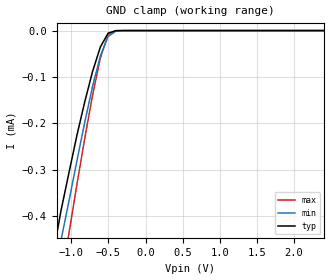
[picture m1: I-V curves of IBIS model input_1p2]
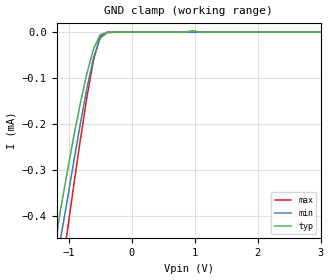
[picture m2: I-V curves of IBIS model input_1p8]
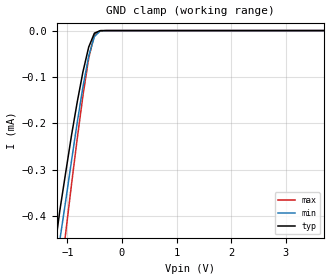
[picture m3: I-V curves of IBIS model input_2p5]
| Texas Instruments Incorporated
| SN74LXC2T45 2-Bit Dual Supply Voltage Translator
| with 3-State outputs and Schmitt-trigger Inputs
[IBIS Ver]   4.1
[File name]   sn74lxc2t45.ibs
[File Rev]   1.0
[Date]   04/24/2019
[Source]
| Texas Instruments Incorporated.
| Analog-eLab Design Center, HPA
| 12500 TI Blvd
| Dallas, TX -75243
[Notes]   Revision History:
| Rev 1.0: 09/01/2020
| - Initial version of the model
| - Model generated from simulations in SPECTRE
| - C_comp although listed in numerical order of value are
|   obtained from varying PVT conditions. For PVT conditions for
|   each specific value refer the buffer description under
|   respective [Model]. IBIS model user is responsible for using
|   appropriate C_comp to simulate for Signal Integrity.
| - Warnings regarding combined Non-monotonicity of various models have been
|   reviewd and considered minor and can be ignored.
| - Model names with a trailing _2p5 contain the model for 2.5V operation.
[Disclaimer]
| This model is designed as an aid for customers of Texas Instruments.
| TI and its licensors and suppliers make no warranties, either expressed
| or implied, with respect to this  model, including the warranties of
| merchantability or fitness for a particular purpose. The model is
| provided solely on an "as is" basis. The entire risk as to its quality
| and performance is with the customer.
| This model is subject to change without notice. Texas Instruments
| Incorporated is not responsible for updating this model.
[Copyright]
 (C) Copyright 2020 Texas Instruments Incorporated.All rights reserved.
| Component LXC2T45_DCT 8-pin SOT
[Component]   SN74LXC2T45DCT
[Manufacturer]   Texas Instruments, Inc.
[Package]
|   typ   min   max
R_pkg   2.900e-02   2.800e-02   3.100e-02
L_pkg   1.796e-09   1.666e-09   1.924e-09
C_pkg   2.310e-13   2.210e-13   2.420e-13
[Pin]   signal_name   model_name   R_pin   L_pin   C_pin
1   VCCA   power   3.100e-02   1.894e-09   2.230e-13
2   A1   I/O   2.800e-02   1.697e-09   2.370e-13
3   A2   I/O   3.000e-02   1.722e-09   2.390e-13
4   GND   gnd   3.000e-02   1.861e-09   2.210e-13
5   DIR   input   2.800e-02   1.924e-09   2.280e-13
6   B2   I/O   2.900e-02   1.736e-09   2.420e-13
7   B1   I/O   2.800e-02   1.666e-09   2.360e-13
8   VCCB   power   3.000e-02   1.871e-09   2.220e-13
| Component LXC2T45_DCU 8-pin SOT
[Component]   SN74LXC2T45DCU
[Manufacturer]   Texas Instruments, Inc.
[Package]
|   typ   min   max
R_pkg   2.600e-02   2.300e-02   3.800e-02
L_pkg   1.394e-09   1.066e-09   2.046e-09
C_pkg   2.590e-13   2.150e-13   3.720e-13
[Pin]   signal_name   model_name   R_pin   L_pin   C_pin
1   VCCA   power   2.400e-02   1.520e-09   2.710e-13
2   A1   I/O   2.300e-02   1.112e-09   2.180e-13
3   A2   I/O   2.300e-02   1.070e-09   2.170e-13
4   GND   gnd   2.700e-02   2.046e-09   3.720e-13
5   DIR   input   2.700e-02   1.542e-09   2.730e-13
6   B2   I/O   2.300e-02   1.100e-09   2.240e-13
7   B1   I/O   2.300e-02   1.066e-09   2.150e-13
8   VCCB   power   3.800e-02   1.696e-09   2.800e-13
|Component
[Component]   SN74LXC2T45DTM
[Manufacturer]  TI
[Package]   |  8 pin  X2SON
|   typ   min   max
R_pkg   0.05   0.04   0.06
L_pkg   1.0nH   0.8nH   1.2nH
C_pkg   0.2pF   0.16pF   0.24pF
[Pin]  signal_name model_name   R_pin   L_pin   C_pin
1   VCCA   power   NA   NA   NA
2   A1   I/O   NA   NA   NA
3   A2   I/O   NA   NA   NA
4   GND   gnd   NA   NA   NA
5   DIR   input   NA   NA   NA
6   B2   I/O   NA   NA   NA
7   B1   I/O   NA   NA   NA
8   VCCB   power   NA   NA   NA
|Component
[Component]   SN74LXC2T45DTT
[Manufacturer]  TI
[Package]   |  8 pin  VQFN
|   typ   min   max
R_pkg   0.05   0.04   0.06
L_pkg   1.0nH   0.8nH   1.2nH
C_pkg   0.2pF   0.16pF   0.24pF
[Pin]  signal_name model_name   R_pin   L_pin   C_pin
1   VCCA   power   NA   NA   NA
2   A1   I/O   NA   NA   NA
3   A2   I/O   NA   NA   NA
4   GND   gnd   NA   NA   NA
5   DIR   input   NA   NA   NA
6   B2   I/O   NA   NA   NA
7   B1   I/O   NA   NA   NA
8   VCCB   power   NA   NA   NA
|   Model Selectors
[Model Selector] input
input_1p2   1.2V   digital input
input_1p8   1.8V   digital input
input_2p5   2.5V   digital input
input_3p3   3.3V   digital input
input_5p0   5.0V   digital input
[Model Selector] I/O
io_1p2   1.2V   Vcc
io_1p8   1.8V   Vcc
io_2p5   2.5V   Vcc
io_3p3   3.3V   Vcc
io_5p0   5.0V   Vcc
| Models and submodels in the file (10): input_1p2 (Input), input_1p8 (Input), input_2p5 (Input), input_3p3 (Input), input_5p0 (Input), io_1p2 (I/O), io_1p8 (I/O), io_2p5 (I/O), io_3p3 (I/O), io_5p0 (I/O)
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|   input_1p2 Model
[Model]   input_1p2
Model_type   Input
Vinl = 0.2
Vinh = 0.9
|   typ   min   max
C_comp   0.119pF   0.105pF   0.126pF
[Voltage Range]   1.2   1.08   1.32
|Junction Temperature
[Temperature Range]   25   125   -40
[GND Clamp Reference]   0   0   0
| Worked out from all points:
|   GND clamp passes 1 mA (typ) near -1.81 V on its own axis
[GND Clamp]
|   Voltage   I(typ)   I(min)   I(max)
-2.5V     -1.66mA    -1.64mA    -2.09mA
-1.24V    -478uA     -541uA     -650uA
-1.14V    -389uA     -453uA     -542uA
-1.03V    -305uA     -366uA     -435uA
-925mV    -226uA     -281uA     -332uA
-820mV    -154uA     -198uA     -233uA
-715mV    -88.7uA    -121uA     -140uA
-610mV    -35.6uA    -54.9uA    -59.7uA
-505mV    -5.5uA     -12.7uA    -8.49uA
-400mV    -210nA     -1.13uA    -141nA
8V        3.62nA     3.43nA     4.23nA
|   input_1p8 Model
[Model]   input_1p8
Model_type   Input
Vinl = 0.7
Vinh = 1.1
|   typ   min   max
C_comp   3.13pF   2.65pF   3.82pF
| Where Nom  PVT is Nominal Process, 2.25V, 27C
|   Fast PVT is Strong Process,  2.50V, -55C
|   Slow PVT is Weak Process,   2.0V, 150C
[Voltage Range]   1.8   1.62   1.98
|Junction Temperature
[Temperature Range]   25   125   -40
[GND Clamp Reference]   0   0   0
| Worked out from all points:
|   GND clamp passes 1 mA (typ) near -1.81 V on its own axis
[GND Clamp]
|   Voltage   I(typ)   I(min)   I(max)
-2.5V     -1.66mA    -1.64mA    -2.09mA
-1.24V    -478uA     -541uA     -650uA
-1.14V    -389uA     -453uA     -542uA
-1.03V    -305uA     -366uA     -435uA
-820mV    -154uA     -198uA     -233uA
-715mV    -88.7uA    -121uA     -140uA
-610mV    -35.6uA    -54.9uA    -59.7uA
-505mV    -5.5uA     -12.7uA    -8.49uA
-400mV    -210nA     -1.13uA    -141nA
965mV     3.74uA     3.02nA     4.93nA
1.07V     3.25nA     2.95nA     3.92nA
8V        3.62nA     3.43nA     4.23nA
|   input_2p5 Model
[Model]   input_2p5
Model_type   Input
Vinl = 1.0
Vinh = 1.4
|   typ   min   max
C_comp   3.03pF   2.54pF   3.83pF
| Where Nom  PVT is Nominal Process, 2.25V, 27C
|   Fast PVT is Strong Process,  2.50V, -55C
|   Slow PVT is Weak Process,   2.0V, 150C
[Voltage Range]   2.5   2.25   2.75
|Junction Temperature
[Temperature Range]   25   125   -40
[GND Clamp Reference]   0   0   0
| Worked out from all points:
|   GND clamp passes 1 mA (typ) near -1.81 V on its own axis
[GND Clamp]
|   Voltage   I(typ)   I(min)   I(max)
-2.5V     -1.66mA    -1.64mA    -2.09mA
-1.24V    -478uA     -541uA     -650uA
-1.14V    -389uA     -453uA     -542uA
-1.03V    -305uA     -366uA     -435uA
-925mV    -226uA     -281uA     -332uA
-820mV    -154uA     -198uA     -233uA
-715mV    -88.7uA    -121uA     -140uA
-610mV    -35.6uA    -54.9uA    -59.7uA
-505mV    -5.5uA     -12.7uA    -8.49uA
-400mV    -210nA     -1.14uA    -141nA
8V        3.62nA     3.43nA     4.23nA
